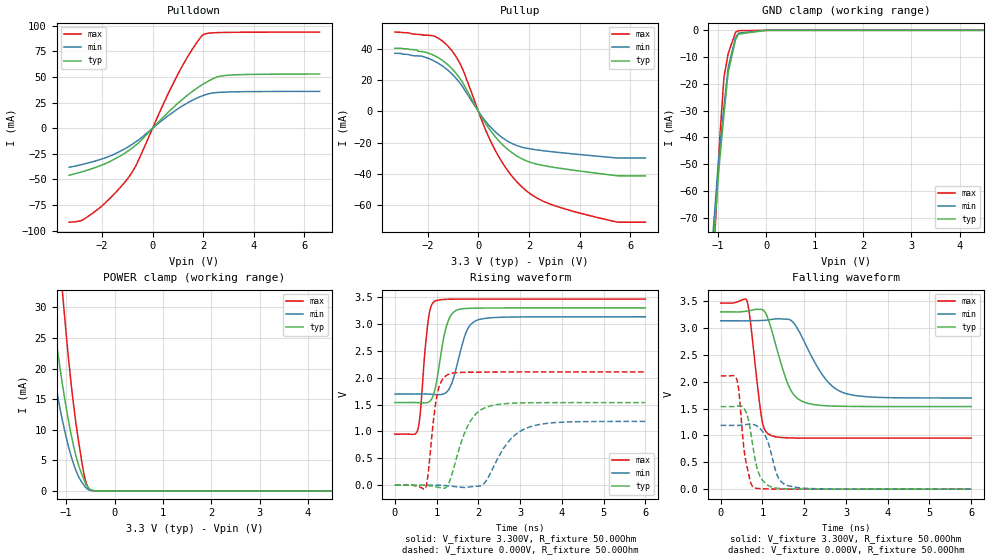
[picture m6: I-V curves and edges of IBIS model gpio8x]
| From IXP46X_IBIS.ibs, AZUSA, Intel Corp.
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[Model]   gpio8x
Model_type   I/O
Vinl = 800.000mV
Vinh = 2.000V
Vmeas = 1.500V
Cref = 0.000F
|   typ   min   max
C_comp   3.000pF   2.700pF   3.300pF
[Voltage Range]   3.300V   3.135V   3.465V
[Temperature Range]   25.0   110.0   -40.0
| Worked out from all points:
|   slope of the pulldown table from 0 to 0.495 V, typ, clamps not added: 39.3 ohm
|   slope of the pullup table from 0 to 0.495 V, typ, clamps not added: 39 ohm
|   POWER clamp passes 1 mA (typ) near -0.59 V on its own axis
|   falling waveform, V_fixture 3.300V, R_fixture 50.00Ohm: 20-80 % time 424ps typ, 647ps min, 221ps max; typ from 3.3 V to 1.54 V
|   rising waveform, V_fixture 3.300V, R_fixture 50.00Ohm: 20-80 % time 241ps typ, 307ps min, 161ps max; typ from 1.54 V to 3.3 V
|   rising waveform, V_fixture 0.000V, R_fixture 50.00Ohm: 20-80 % time 435ps typ, 607ps min, 189ps max; typ from 0 V to 1.54 V
|   falling waveform, V_fixture 0.000V, R_fixture 50.00Ohm: 20-80 % time 228ps typ, 272ps min, 177ps max; typ from 1.54 V to 0 V
[Pulldown]
|   Voltage   I(typ)   I(min)   I(max)
-3.3V     -45.91mA   -38.12mA   -91.69mA
-2.81V    -42.66mA   -35.52mA   -89.99mA
-2.26V    -38.3mA    -31.96mA   -80.93mA
-1.595V   -31.33mA   -26.29mA   -66.18mA
-925mV    -21.49mA   -17.59mA   -47.13mA
-605mV    -15.45mA   -12.4mA    -33.74mA
370mV     9.528mA    7.525mA    20.66mA
985mV     24mA       18.65mA    51.97mA
1.535V    35.18mA    26.77mA    75.76mA
1.99V     42.89mA    31.83mA    90.98mA
2.875V    51.45mA    35.27mA    93.44mA
6.595V    52.88mA    35.95mA    93.77mA
[GND Clamp]
|   Voltage   I(typ)   I(min)   I(max)
-3.3V     -1.837A    -1.782A    -2.189A
-1.11V    -84.95mA   -77.98mA   -94.01mA
-995mV    -55.64mA   -50.79mA   -51.59mA
-965mV    -49.2mA    -44.86mA   -41.53mA
-875mV    -31.64mA   -28.58mA   -17.71mA
-790mV    -16.2mA    -14.47mA   -9.012mA
-785mV    -15.56mA   -13.64mA   -8.605mA
-635mV    -3.546mA   -2.727mA   -731.7uA
-575mV    -1.513mA   -1.11mA    -135.3uA
0V        -56.84nA   -17.58nA   -65.5pA
6.595V    0A         0A         0A
[Pullup]
|   Voltage   I(typ)   I(min)   I(max)
-3.3V     40.55mA    37.31mA    50.89mA
-1.775V   36.07mA    32.58mA    48.46mA
-1.065V   27.72mA    24.33mA    39.28mA
-630mV    18.64mA    16.01mA    27.31mA
215mV     -5.981mA   -4.928mA   -9.158mA
695mV     -16.78mA   -13.51mA   -25.89mA
1.25V     -25.55mA   -19.92mA   -39.99mA
1.945V    -32.03mA   -23.75mA   -51.58mA
2.78V     -35.34mA   -25.63mA   -59.11mA
3.83V     -37.88mA   -27.39mA   -64.5mA
5.5V      -41.29mA   -29.89mA   -71.03mA
6.595V    -41.3mA    -29.89mA   -71.04mA
[POWER Clamp]
|   Voltage   I(typ)   I(min)   I(max)
-3.3V     221.1mA    178.3mA    361mA
-1.505V   44.7mA     32.22mA    80.58mA
-1.325V   32.02mA    22.46mA    58.62mA
-1.2V     24.19mA    16.55mA    44.79mA
-1.08V    17.53mA    11.61mA    32.8mA
-1.04V    15.51mA    10.14mA    29.12mA
-910mV    9.707mA    6.02mA     18.41mA
-800mV    5.804mA    3.374mA    11.15mA
-640mV    2mA        1.037mA    3.043mA
-540mV    479.4uA    207uA      465.4uA
-395mV    31.37uA    12.42uA    6.173uA
6.595V    0A         0A         0A
[Ramp]
R_load = 50.00Ohm
|   typ   min   max
dV/dt_r   922.440mV/434.659ps 712.650mV/605.447ps   1.265V/188.348ps
dV/dt_f   1.057V/423.874ps 862.881mV/645.791ps   1.509V/220.628ps
[Falling Waveform]
V_fixture = 3.300V
V_fixture_min = 3.135V
V_fixture_max = 3.465V
R_fixture = 50.00Ohm
|   Time   V(typ)   V(min)   V(max)
0s        3.3V       3.135V     3.465V
630ps     3.315V     3.134V     3.503V
710ps     3.327V     3.135V     3.126V
980ps     3.345V     3.14V      1.322V
1.17ns    3.088V     3.154V     1.012V
1.63ns    1.921V     3.161V     954.8mV
1.97ns    1.629V     2.795V     951mV
2.48ns    1.555V     2.081V     950.9mV
2.92ns    1.543V     1.801V     951.2mV
6ns       1.538V     1.697V     949.8mV
[Rising Waveform]
V_fixture = 3.300V
V_fixture_min = 3.135V
V_fixture_max = 3.465V
R_fixture = 50.00Ohm
|   Time   V(typ)   V(min)   V(max)
0s        1.538V     1.697V     949.8mV
550ps     1.537V     1.697V     1.037V
610ps     1.534V     1.698V     1.359V
800ps     1.545V     1.696V     3.078V
960ps     1.784V     1.688V     3.427V
1.23ns    2.946V     1.726V     3.46V
1.49ns    3.261V     2.243V     3.464V
1.74ns    3.291V     2.903V     3.465V
2.01ns    3.297V     3.084V     3.465V
6ns       3.3V       3.135V     3.465V
[Rising Waveform]
V_fixture = 0.000V
V_fixture_min = 0.000V
V_fixture_max = 0.000V
R_fixture = 50.00Ohm
|   Time   V(typ)   V(min)   V(max)
0s        1.225uV    430.3nV    -6.12nV
730ps     -2.357mV   447uV      -59.71mV
790ps     -6.423mV   579.3uV    173.5mV
1.01ns    -34.24mV   108.1uV    1.675V
1.27ns    2.167mV    -10.83mV   2.058V
1.75ns    1.111V     -36.69mV   2.103V
2.16ns    1.442V     52.68mV    2.106V
2.69ns    1.521V     781mV      2.108V
3.16ns    1.533V     1.065V     2.108V
6ns       1.537V     1.188V     2.108V
[Falling Waveform]
V_fixture = 0.000V
V_fixture_min = 0.000V
V_fixture_max = 0.000V
R_fixture = 50.00Ohm
|   Time   V(typ)   V(min)   V(max)
0s        1.537V     1.188V     2.108V
390ps     1.546V     1.186V     2.03V
440ps     1.552V     1.187V     1.784V
590ps     1.462V     1.202V     572.8mV
720ps     1.05V      1.211V     116.8mV
810ps     609.9mV    1.197V     25.95mV
1.06ns    117.4mV    1.003V     6.195mV
1.36ns    17.44mV    245.9mV    1.877mV
1.62ns    6.424mV    62.42mV    406.5uV
6ns       1.225uV    430.3nV    -6.12nV
